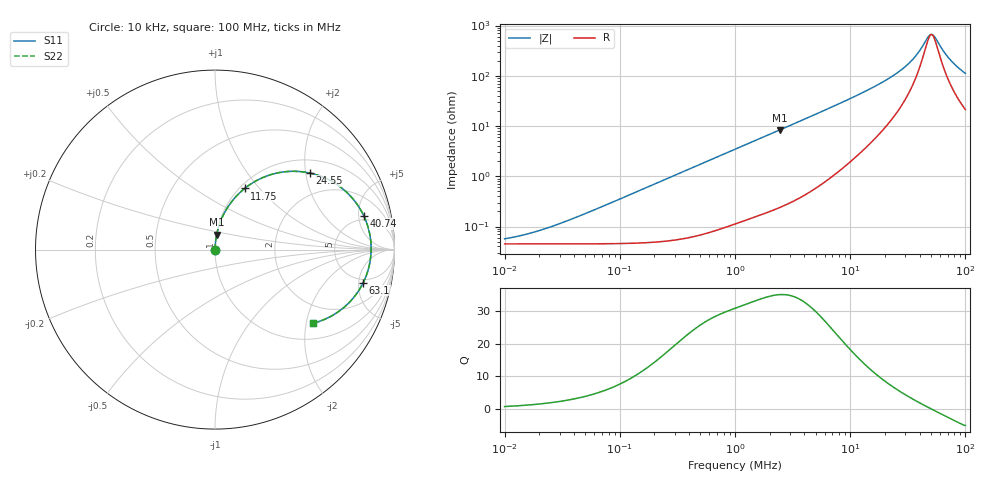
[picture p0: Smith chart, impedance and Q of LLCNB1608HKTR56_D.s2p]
! LLCNB1608HKTR56_D  S-PARAMETER MODEL  ( Standard Model )
! Model Generated by TAIYO YUDEN Corporation (http://www.ty-top.com)
! Version 1.0
! TAIYO YUDEN Control No. 200410
! Copyright(c) 2020 TAIYO YUDEN CO.,LTD. All Rights Reserved.
! Product Description (link to TY-COMPAS)
! https://ds.yuden.co.jp/TYCOMPAS/or/detail?pn=LLCNB1608HKTR56MD&u=M
! Products Name : Inductors
! Characteristics :
!  Inductance : 0.56 [uH] , SRF(min) : - [Hz] , DC Resistance(max) : 55 [mOhm]
!  Rated Current : Saturation  2.7 [A] (dL = 30 [%]), Temp Rise  2.6 [A] (dT = 40 [degC])
!  Case Size : 1.6 x 0.8 / 0.063 x 0.031 [mm/inch] , Thickness : 0.8 / 0.031 [mm/inch]
!  (Conditions: Temperature = 25 [degC] , DC Bias Current = 0 [A])
! External Node Assignments :
!  1  o---GGG---o  2
! GND o---------o GND
! Frequency Range : 10kHz  -  100MHz  [ 402 STEP ]
# MHz S RI R 50
! Freq[MHz].  S11 Real  S11 Imag  S21 Real  S21 Imag  S12 Real  S12 Imag  S22 Real  S22 Imag
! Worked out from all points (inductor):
!   401 points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, 10 kHz to 100 MHz, reference 50 ohm
!   read as one part in series: L = 555 nH near 38.91 kHz
!   highest Q = 35 at 2.455 MHz (marker M1), where L = 544 nH
!   self-resonance near 50.81 MHz
!   S11 on the Smith chart (normalised r, x): 10 kHz: 1.00, +0.00; 11.75 MHz: 1.05, +0.84; 24.55 MHz: 1.33, +2.12; 40.74 MHz: 4.30, +5.83; 63.1 MHz: 4.44, -5.74; 100 MHz: 1.43, -2.19
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0.01  0.00045 0.000348  0.9996 -0.000348  0.9996 -0.000348  0.00045 0.000348
0.019953  0.00045 0.000695  0.9995 -0.000695  0.9995 -0.000695  0.00045 0.000695
0.046774  0.000453 0.00163  0.9995 -0.00163  0.9995 -0.00163  0.000453 0.00163
0.218776  0.000553 0.00763  0.9994 -0.00763  0.9994 -0.00763  0.000553 0.00763
1  0.0023 0.0344  0.9977 -0.0344  0.9977 -0.0344  0.0023 0.0344
2.454709  0.00932 0.0829  0.9907 -0.0829  0.9907 -0.0829  0.00932 0.0829
4.677351  0.0298 0.1545  0.9702 -0.1545  0.9702 -0.1545  0.0298 0.1545
7.762471  0.0771 0.2455  0.9229 -0.2455  0.9229 -0.2455  0.0771 0.2455
11.74898  0.1653 0.3408  0.8347 -0.3408  0.8347 -0.3408  0.1653 0.3408
16.2181  0.2878 0.4098  0.7122 -0.4098  0.7122 -0.4098  0.2878 0.4098
21.87762  0.4544 0.436  0.5456 -0.436  0.5456 -0.436  0.4544 0.436
24.54709  0.5295 0.4265  0.4705 -0.4265  0.4705 -0.4265  0.5295 0.4265
32.35937  0.7126 0.3379  0.2874 -0.3379  0.2874 -0.3379  0.7126 0.3379
36.30781  0.7781 0.2708  0.2219 -0.2708  0.2219 -0.2708  0.7781 0.2708
40.73803  0.8292 0.1877  0.1708 -0.1877  0.1708 -0.1877  0.8292 0.1877
47.86301  0.8672 0.0527  0.1328 -0.0527  0.1328 -0.0527  0.8672 0.0527
51.28614  0.8696 -0.00823  0.1304 0.00823  0.1304 0.00823  0.8696 -0.00823
54.95409  0.8634 -0.0689  0.1366 0.0689  0.1366 0.0689  0.8634 -0.0689
63.09573  0.8262 -0.1836  0.1738 0.1836  0.1738 0.1836  0.8262 -0.1836
69.1831  0.7852 -0.251  0.2148 0.251  0.2148 0.251  0.7852 -0.251
77.62471  0.7197 -0.3211  0.2803 0.3211  0.2803 0.3211  0.7197 -0.3211
100  0.546 -0.41  0.454 0.41  0.454 0.41  0.546 -0.41
